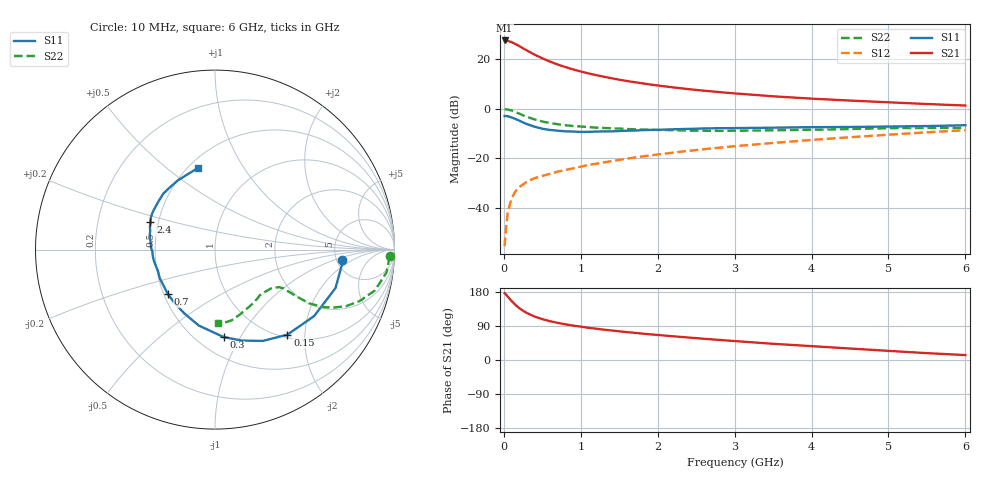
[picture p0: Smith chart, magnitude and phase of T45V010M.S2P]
! Infineon Technologies  Discrete & RF Semiconductors
! BFR182T
! Si NPN RF Bipolar Junction Transistor in SC75
! VCE = 5 V  IC = 10 mA
! Common Emitter S-Parameters:  October  1999
# GHz  S  MA  R  50
!  f  S11  S21  S12  S22
! GHz  MAG  ANG  MAG  ANG  MAG  ANG  MAG  ANG
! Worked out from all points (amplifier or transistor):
!   36 points, 10 MHz to 6 GHz, reference 50 ohm
!   highest |S21| = 27.5 dB at 10 MHz (marker M1)
!   |S21| within 3 dB of that: start of sweep to 241.4 MHz
!   unconditionally stable (mu >= 1): 1.072 GHz to 3.838 GHz
!   at 250 MHz: K = 0.44, MSG = 27.4 dB, |S12| = -30.5 dB
!   at 1.4 GHz: K = 1.06, MAG = 15.2 dB, |S12| = -21.1 dB
!   at 6 GHz: K = 0.85, MSG = 5.0 dB, |S12| = -8.6 dB
!   lowest NFmin = 1.50 dB at 450 MHz
!   S11 on the Smith chart (normalised r, x): 10 MHz: 5.56, -1.24; 150 MHz: 1.06, -1.63; 300 MHz: 0.67, -0.85; 700 MHz: 0.52, -0.30; 2.4 GHz: 0.45, +0.17; 6 GHz: 0.56, +0.65
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0.01  0.708 -4.5  23.68 176.3  0.0017 73.0  0.9739 -2.2
0.02  0.7143 -5.7  23.6 174.9  0.0029 98.1  0.9721 -3.0
0.05  0.7047 -17.7  23.27 167.2  0.0081 84.1  0.9638 -7.6
0.1  0.6651 -33.8  21.89 155.9  0.0154 76.9  0.9197 -14.3
0.15  0.6223 -49.6  20.14 145.5  0.0216 69.9  0.8551 -19.6
0.2  0.5746 -62.3  18.3 137.0  0.0264 66.5  0.7945 -23.4
0.25  0.5283 -73.6  16.46 129.9  0.0298 61.5  0.7339 -26.1
0.3  0.4899 -84.3  14.85 123.9  0.034 61.1  0.6853 -27.9
0.4  0.433 -101.9  12.27 114.5  0.0398 58.6  0.6054 -29.7
0.5  0.3953 -115.4  10.34 107.8  0.0442 58.9  0.5526 -29.8
0.6  0.3729 -127.4  8.866 102.4  0.0488 58.8  0.5144 -29.9
0.7  0.3606 -137.0  7.767 98.0  0.0541 60.5  0.4861 -29.7
0.9  0.3468 -152.7  6.184 90.9  0.0628 62.2  0.4477 -29.6
1.1  0.342 -164.7  5.143 85.0  0.0737 63.4  0.4258 -30.0
1.3  0.3488 -174.2  4.405 80.1  0.083 64.4  0.4086 -30.9
1.6  0.3605 174.8  3.613 73.6  0.0986 65.5  0.3901 -32.7
2.2  0.3842 160.6  2.686 62.6  0.1304 66.1  0.3683 -38.7
2.4  0.3915 156.7  2.477 59.3  0.1414 66.0  0.3621 -41.2
3.5  0.4143 139.3  1.776 42.8  0.2043 63.2  0.3672 -55.4
4.5  0.428 126.2  1.457 30.3  0.266 58.9  0.3891 -69.9
5.5  0.4466 109.9  1.243 18.1  0.3339 53.6  0.4099 -82.4
6  0.4643 101.9  1.157 13.0  0.3695 50.1  0.4106 -87.5
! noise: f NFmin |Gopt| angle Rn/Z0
0.45  1.5  0.26  43  0.28
0.9  1.6  0.24  87  0.22
1.8  2.1  0.2  170  0.2
